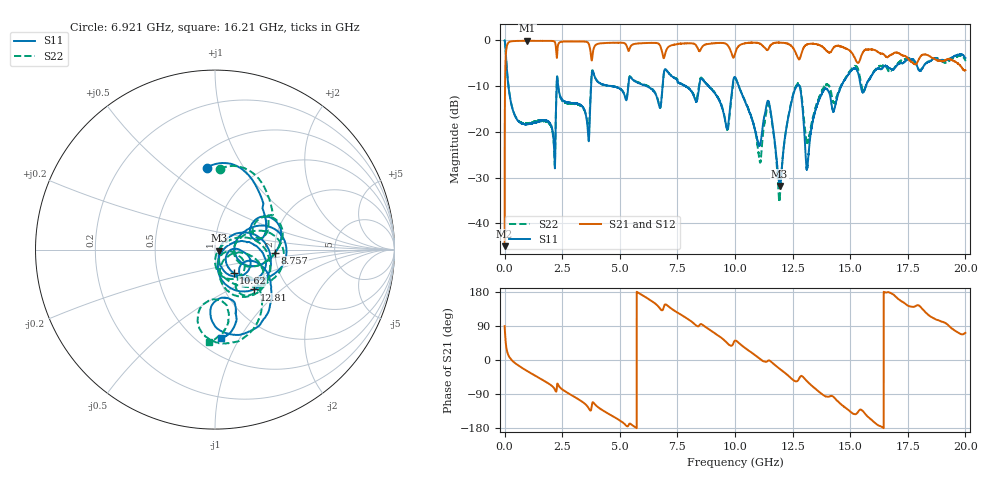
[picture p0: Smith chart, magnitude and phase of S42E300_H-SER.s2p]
! Created Wed Nov 25 22:09:44 2020
# khz S ma R 50
! 2 Port Network Data from SP1.SP block
! freq  magS11  angS11  magS21  angS21  magS12  angS12  magS22  angS22
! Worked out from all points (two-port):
!   20001 points, 300 kHz to 20 GHz, reference 50 ohm
!   highest |S21| = -0.08 dB at 982.3 MHz (marker M1); lowest = -45.0 dB at 300 kHz (marker M2)
!   |S21| within 3 dB of the highest: 3.82 GHz to 6.859 GHz (3.039 GHz wide, 56.9 % of centre); 6.961 GHz to 9.869 GHz (2.908 GHz wide, 34.6 % of centre)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
!   lowest |S11| = -31.8 dB at 11.94 GHz (marker M3), VSWR 1.05, Z = 52.5 - j0.681 ohm
!   |S11| at or under -10 dB: 166.8 MHz to 2.258 GHz (2.091 GHz wide, 172 % of centre); 10.17 GHz to 12.67 GHz (2.508 GHz wide, 22 % of centre); 12.8 GHz to 14.61 GHz (1.803 GHz wide, 13.2 % of centre)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
!   |S22| runs from -34.9 to 0.0 dB; largest |S21 - S12| = 0.018
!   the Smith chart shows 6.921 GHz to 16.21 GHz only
!   S11 on the Smith chart (normalised r, x): 6.921 GHz: 0.61, +0.70; 8.757 GHz: 2.01, -0.07; 10.62 GHz: 1.18, -0.32; 12.81 GHz: 1.36, -0.67; 16.21 GHz: 0.64, -0.84
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300  0.9989 -0.5  0.005644 89.3  0.005608 88.7  0.9978 -0.3
134300  0.3788 -72.7  0.924 17.3  0.9246 17.2  0.3803 -72.8
982300  0.1216 -121.1  0.9908 -29.2  0.9892 -29.2  0.1242 -119.0
3334300  0.1941 158.0  0.9737 -108.8  0.9726 -108.7  0.1908 166.2
3859300  0.4386 167.9  0.8046 -112.6  0.8055 -112.6  0.4413 170.3
5129300  0.2769 107.7  0.9427 -164.9  0.9426 -164.9  0.2795 108.2
6667300  0.2137 69.3  0.9258 141.5  0.9245 141.5  0.218 60.0
6921300  0.4574 95.6  0.6454 142.0  0.6458 141.9  0.4494 86.4
8757300  0.3356 -2.8  0.9083 85.7  0.909 85.7  0.338 -2.2
9657300  0.1084 -0.5  0.8998 44.9  0.9025 45.0  0.1066 -8.3
1.00003e7  0.398 -5.4  0.7135 51.2  0.7151 51.3  0.3881 -11.4
1.06183e7  0.1662 -51.5  0.942 23.9  0.9449 23.8  0.1701 -70.2
1.10753e7  0.07126 -19.2  0.9247 3.1  0.9265 3.2  0.04763 -48.0
1.14863e7  0.2041 -46.8  0.8393 -1.3  0.8394 -1.2  0.1912 -58.9
1.19363e7  0.02571 -14.6  0.9461 -23.2  0.9484 -23.1  0.01825 -18.0
1.28133e7  0.31 -45.8  0.6331 -45.8  0.6364 -45.9  0.3252 -52.2
1.31133e7  0.03953 -38.0  0.9006 -55.1  0.9001 -55.2  0.0765 -52.3
1.33343e7  0.1147 20.9  0.9192 -67.9  0.9198 -67.8  0.1281 -7.5
1.62113e7  0.4939 -86.2  0.747 -172.1  0.7414 -172.0  0.5142 -93.8
1.66673e7  0.5028 -103.3  0.6699 179.1  0.6571 179.0  0.461 -117.2
1.83893e7  0.5814 -148.6  0.6863 119.2  0.6857 119.7  0.5894 -155.7
2e7  0.6443 155.6  0.4752 71.8  0.4769 72.6  0.6006 137.5
